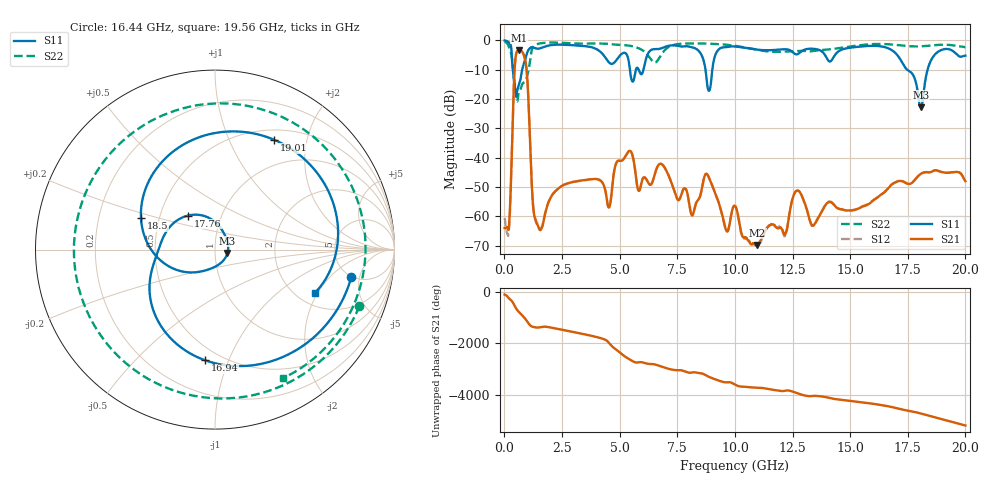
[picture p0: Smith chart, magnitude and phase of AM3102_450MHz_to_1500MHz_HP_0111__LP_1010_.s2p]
!Agilent Technologies,E8364B,MY43040894,A.07.50.67
!Agilent E8364B: A.07.50.67
!Date: Thursday, January 11, 2018 05:53:40
!Correction: S11(Full 2 Port(1,2))
!S21(Full 2 Port(1,2))
!S12(Full 2 Port(1,2))
!S22(Full 2 Port(1,2))
!S2P File: Measurements: S11, S21, S12, S22:
# Hz S  dB  R 50
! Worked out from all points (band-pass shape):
!   1601 points, 10 MHz to 20 GHz, reference 50 ohm
!   highest |S21| = -3.35 dB at 634.7 MHz (marker M1); lowest = -69.8 dB at 10.98 GHz (marker M2)
!   |S21| within 3 dB of the highest: 478.5 MHz to 893.8 MHz (415.2 MHz wide, 60.5 % of centre)
!   lowest |S11| = -22.8 dB at 18.06 GHz (marker M3), VSWR 1.16, Z = 57.4 - j2.21 ohm
!   |S11| at or under -10 dB: 366.4 MHz to 772.3 MHz (405.8 MHz wide, 71.3 % of centre); 8.724 GHz to 9.02 GHz (296.1 MHz wide, 3.34 % of centre); 17.47 GHz to 18.36 GHz (890.1 MHz wide, 4.97 % of centre)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
!   |S22| runs from -20.9 to -0.5 dB; largest |S21 - S12| = 0.0015
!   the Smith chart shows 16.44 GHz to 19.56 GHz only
!   S11 on the Smith chart (normalised r, x): 16.44 GHz: 4.91, -3.78; 16.94 GHz: 0.41, -0.83; 17.76 GHz: 0.69, +0.28; 18.5 GHz: 0.39, +0.17; 19.01 GHz: 0.63, +1.49; 19.56 GHz: 2.49, -1.89
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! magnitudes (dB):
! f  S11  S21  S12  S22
! 10 MHz  -0.1  -64.0  -60.5  -0.5
! 197.4 MHz  -0.7  -63.7  -64.4  -2.3
! 459.8 MHz  -16.2  -8.0  -8.0  -15.3
! 634.7 MHz  -15.1  -3.3  -3.4  -17.5
! 934.5 MHz  -5.6  -8.0  -8.0  -13.5
! 1.459 GHz  -2.9  -63.2  -63.1  -1.2
! 3.346 GHz  -1.9  -47.8  -47.8  -1.1
! 6.682 GHz  -3.0  -42.6  -42.5  -6.5
! 8.881 GHz  -17.2  -46.9  -46.9  -1.2
! 10.01 GHz  -2.1  -56.5  -56.4  -1.9
! 10.98 GHz  -3.2  -69.8  -70.2  -3.3
! 12.69 GHz  -4.8  -51.2  -51.3  -3.6
! 13.34 GHz  -2.9  -63.2  -63.1  -3.7
! 16.44 GHz  -2.2  -52.1  -52.2  -1.3
! 16.68 GHz  -2.8  -50.2  -50.1  -1.4
! 16.94 GHz  -4.2  -48.5  -48.5  -1.6
! 17.76 GHz  -12.3  -48.0  -47.9  -2.1
! 18.06 GHz  -22.8  -45.6  -45.5  -2.1
! 18.5 GHz  -7.0  -44.9  -44.9  -1.8
! 19.01 GHz  -3.2  -45.0  -45.0  -1.5
! 19.56 GHz  -4.3  -44.9  -44.9  -1.8
! 20 GHz  -5.2  -48.0  -48.0  -2.3
